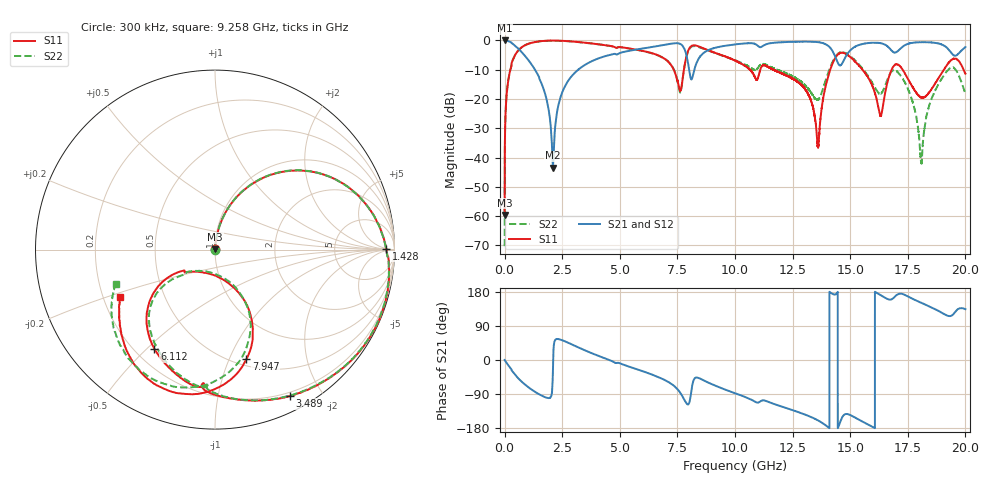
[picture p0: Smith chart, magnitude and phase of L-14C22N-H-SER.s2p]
!{L-14C22N}
!Johanson Technology Inc.
!www.johansontechnology.com
!Test Board Conditions:
!Substrate Type  RO4350B
!Substrate Thickness  20 mil
!Substrate Dk  3.66
!TL Type: GCPW
!TL Trace Width  36 mil
!TL Gap  12 mil
!Electrode orientation  Horizontal
!DUT TOPOLOGY	SERIES
!Mounting Pad LxW  26x36 mil
! Created Sun Jun 20 13:03:03 2021
# hz S ma R 50
! 2 Port Network Data from SP1.SP block
! freq  magS11  angS11  magS21  angS21  magS12  angS12  magS22  angS22
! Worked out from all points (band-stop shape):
!   20001 points, 300 kHz to 20 GHz, reference 50 ohm
!   highest |S21| = 0.00 dB at 300 kHz (marker M1); lowest = -43.5 dB at 2.097 GHz (marker M2)
!   |S21| within 3 dB of the highest: 8.938 GHz to 14.18 GHz (5.246 GHz wide, 45.4 % of centre); 17.15 GHz to 19.26 GHz (2.108 GHz wide, 11.6 % of centre)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
!   lowest |S11| = -59.7 dB at 300 kHz (marker M3), VSWR 1.00, Z = 50 + j0.103 ohm
!   |S11| at or under -10 dB: 11.68 GHz to 14.13 GHz (2.45 GHz wide, 19 % of centre); 15.54 GHz to 16.8 GHz (1.262 GHz wide, 7.8 % of centre); 17.28 GHz to 19.07 GHz (1.793 GHz wide, 9.87 % of centre)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
!   |S22| runs from -70.3 to -0.1 dB; largest |S21 - S12| = 0.012
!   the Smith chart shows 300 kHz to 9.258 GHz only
!   S11 on the Smith chart (normalised r, x): 300 kHz: 1.00, +0.00; 1.428 GHz: 41, +5; 3.489 GHz: 0.16, -1.62; 6.112 GHz: 0.28, -0.53; 7.947 GHz: 0.57, -1.16; 9.258 GHz: 0.27, -0.22
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300000  0.001038 85.2  0.9999 -0.1  0.9984 -0.0  0.0003056 115.0
1.073e8  0.1424 78.7  0.9848 -9.3  0.9848 -9.4  0.1434 78.7
2.723e8  0.3407 66.1  0.9339 -22.9  0.9336 -22.9  0.3426 66.1
1.4283e9  0.9535 0.4  0.2668 -88.1  0.2679 -88.1  0.9535 0.2
2.0973e9  0.9947 -22.2  0.006701 -24.1  0.0067 -24.4  0.9915 -22.5
3.3343e9  0.93 -58.8  0.3487 29.6  0.3498 29.6  0.9257 -59.2
3.4893e9  0.9153 -63.0  0.3825 25.4  0.3832 25.5  0.9113 -63.5
6.1123e9  0.6475 -121.5  0.742 -32.1  0.7447 -32.1  0.644 -119.2
6.6673e9  0.5558 -133.2  0.8063 -45.0  0.808 -44.9  0.5537 -131.5
7.6113e9  0.1406 -112.5  0.8755 -85.4  0.8768 -85.4  0.1305 -109.8
7.9473e9  0.6348 -74.0  0.4423 -117.3  0.443 -116.9  0.6183 -76.0
9.2583e9  0.5911 -153.2  0.7689 -70.6  0.7725 -70.9  0.5868 -160.9
1.00003e10  0.4534 -170.1  0.8557 -87.8  0.8582 -87.7  0.4597 -177.1
1.33343e10  0.08466 121.2  0.9504 -151.5  0.9501 -151.5  0.1223 153.0
1.36143e10  0.01569 -157.4  0.934 -159.8  0.9354 -159.9  0.0973 -168.1
1.45793e10  0.6109 -175.2  0.3758 -161.6  0.3766 -161.8  0.6283 -177.8
1.63053e10  0.0523 155.6  0.9015 171.9  0.8994 172.1  0.1232 141.2
1.66673e10  0.2272 -147.2  0.7629 159.8  0.7568 160.2  0.2422 159.5
1.74813e10  0.2295 134.5  0.8655 168.6  0.8691 168.7  0.1558 75.9
1.80813e10  0.1068 166.2  0.9317 151.1  0.9357 150.9  0.008032 -48.3
1.91493e10  0.3548 -156.9  0.7784 118.8  0.7832 119.2  0.2833 155.2
2e10  0.2692 132.3  0.769 134.1  0.7651 134.1  0.1189 57.3
